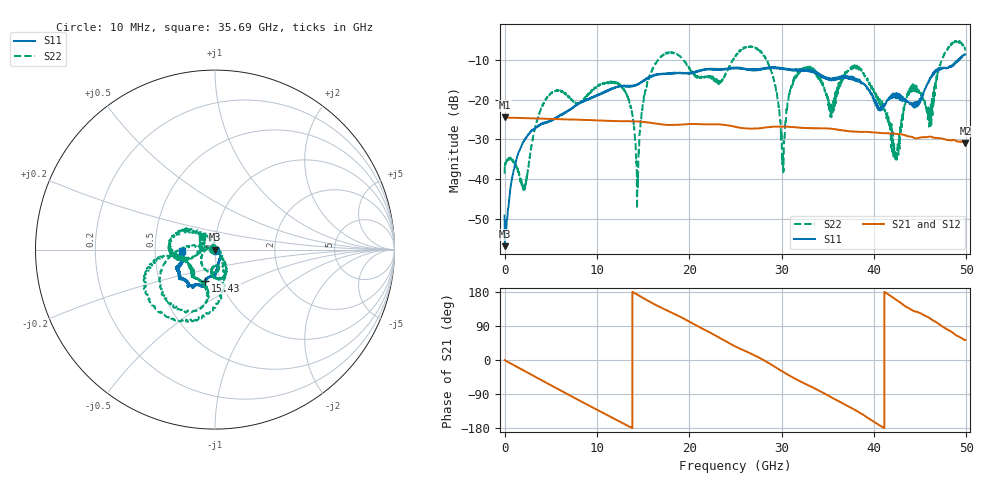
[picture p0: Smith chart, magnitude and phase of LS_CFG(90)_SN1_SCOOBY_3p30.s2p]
!Keysight Technologies,N5245B,MY58422026,A.13.80.08
!Date: Thursday, March 19, 2020 23:55:18
!Correction: S11(Full 2 Port(1,2))
!S21(Full 2 Port(1,2))
!S12(Full 2 Port(1,2))
!S22(Full 2 Port(1,2))
!S2P File: Measurements: S11, S21, S12, S22:
# Hz S DB R 50.0
!freq dBS11 angS11 dBS21 angS21 dBS12 angS12 dBS22 angS22
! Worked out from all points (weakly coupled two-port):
!   4991 points, 10 MHz to 49.91 GHz, reference 50 ohm
!   highest |S21| = -24.49 dB at 10 MHz (marker M1); lowest = -30.9 dB at 49.91 GHz (marker M2)
!   lowest |S11| = -56.9 dB at 30 MHz (marker M3), VSWR 1.00, Z = 50.1 - j0.0226 ohm
!   |S11| at or under -10 dB: start of sweep to 49.12 GHz; 49.16896 GHz to 49.22291 GHz (53.96 MHz wide, 0.11 % of centre)
!   |S22| runs from -47.5 to -5.1 dB; largest |S21 - S12| = 0.0006
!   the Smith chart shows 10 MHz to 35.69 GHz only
!   S11 on the Smith chart (normalised r, x): 10 MHz: 1.00, -0.01; 15.43 GHz: 0.85, -0.30; 35.69 GHz: 0.69, -0.01
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1e7  -49.20 -57.7  -24.49 -0.3  -24.48 -0.3  -38.67 175.3
3e7  -56.91 -9.1  -24.50 -0.5  -24.49 -0.6  -36.52 -174.5
2.15e9  -30.30 -39.4  -24.64 -28.8  -24.63 -28.8  -42.85 36.3
4.51e9  -25.69 -55.0  -24.83 -59.9  -24.82 -59.9  -19.89 -138.0
8.33e9  -20.74 -79.7  -25.07 -109.8  -25.07 -109.7  -20.46 -94.2
1.267e10  -16.66 -90.5  -25.42 -164.6  -25.41 -164.6  -16.59 -67.2
1.437e10  -16.19 -102.3  -25.49 172.7  -25.48 172.8  -42.47 -108.3
1.543e10  -14.83 -107.2  -25.72 157.9  -25.71 158.0  -16.18 172.3
1.665e10  -13.66 -106.8  -26.11 141.8  -26.10 141.9  -9.93 -158.5
2.496e10  -12.08 -127.1  -26.80 36.1  -26.79 36.3  -9.26 -167.7
2.835e10  -12.01 -140.3  -27.00 -4.2  -27.00 -3.9  -9.75 -90.8
3.014e10  -12.22 -144.6  -26.83 -30.8  -26.84 -30.4  -34.48 29.0
3.116e10  -12.44 -147.5  -26.91 -45.2  -26.92 -44.8  -15.81 142.4
3.328e10  -12.82 -156.6  -27.18 -71.6  -27.18 -71.1  -12.15 -174.2
3.569e10  -14.67 -177.4  -27.45 -102.1  -27.39 -101.6  -19.72 135.4
3.816e10  -15.36 176.0  -28.08 -134.6  -28.03 -134.7  -11.42 -175.2
4.16e10  -19.59 105.3  -28.47 172.6  -28.50 172.6  -25.11 69.9
4.245e10  -18.60 104.7  -28.63 158.5  -28.65 158.4  -34.92 -174.0
4.39e10  -20.84 76.1  -29.28 134.7  -29.29 134.8  -17.45 -32.1
4.601e10  -15.30 5.7  -29.29 110.9  -29.32 111.0  -23.27 114.8
4.771e10  -12.00 5.6  -29.99 83.6  -30.00 83.8  -8.15 -79.7
4.991e10  -8.60 -14.2  -30.89 52.7  -30.91 52.8  -7.33 -14.9
